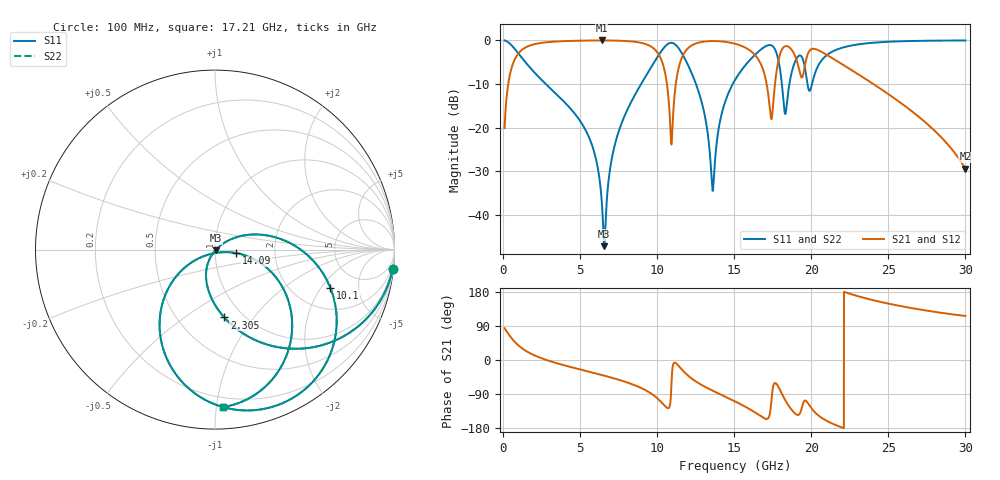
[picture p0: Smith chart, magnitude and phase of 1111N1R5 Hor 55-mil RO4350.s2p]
# GHz S MA R 50
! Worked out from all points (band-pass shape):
!   3201 points, 100 MHz to 30 GHz, reference 50 ohm
!   highest |S21| = -0.04 dB at 6.388 GHz (marker M1); lowest = -29.4 dB at 30 GHz (marker M2)
!   |S21| within 3 dB of the highest: 990.4 MHz to 10.07 GHz (9.075 GHz wide, 164 % of centre); 11.73 GHz to 16.26 GHz (4.523 GHz wide, 32.3 % of centre)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
!   lowest |S11| = -47.1 dB at 6.566 GHz (marker M3), VSWR 1.01, Z = 50.3 - j0.308 ohm
!   |S11| at or under -10 dB: 2.772 GHz to 8.957 GHz (6.185 GHz wide, 105 % of centre); 12.52 GHz to 14.91 GHz (2.388 GHz wide, 17.4 % of centre); 18.09 GHz to 18.58 GHz (487.3 MHz wide, 2.66 % of centre)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
!   |S22| runs from -47.1 to 0.0 dB; largest |S21 - S12| = 0
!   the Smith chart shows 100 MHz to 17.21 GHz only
!   S11 on the Smith chart (normalised r, x): 100 MHz: 1, -18; 2.305 GHz: 0.82, -0.73; 10.1 GHz: 3.13, -2.46; 14.09 GHz: 1.27, -0.05; 17.21 GHz: 0.14, -1.05
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0.1  0.9951 -6.3  0.09907 83.7  0.09907 83.7  0.9951 -6.3
0.7447187  0.8017 -41.5  0.5969 48.5  0.5969 48.5  0.8017 -41.5
2.305125  0.3818 -82.2  0.9223 7.6  0.9223 7.6  0.3818 -82.2
5.089563  0.1131 -114.3  0.9899 -25.9  0.9899 -25.9  0.1131 -114.3
6.388344  0.01562 -113.7  0.9949 -39.4  0.9949 -39.4  0.01562 -113.7
6.565875  0.00443 -43.7  0.9948 -41.3  0.9948 -41.3  0.00443 -43.7
7.472219  0.08737 34.4  0.9894 -51.7  0.9894 -51.7  0.08737 34.4
10.06978  0.6651 -17.1  0.7024 -103.3  0.7024 -103.3  0.6651 -17.1
10.09781  0.6769 -18.3  0.6897 -104.4  0.6897 -104.4  0.6769 -18.3
10.92941  0.9345 -66.9  0.06459 -61.4  0.06459 -61.4  0.9345 -66.9
11.84509  0.5926 -120.3  0.754 -35.3  0.754 -35.3  0.5926 -120.3
13.58303  0.01963 -94.7  0.9795 -80.7  0.9795 -80.7  0.01963 -94.7
14.08759  0.121 -9.3  0.9727 -90.5  0.9727 -90.5  0.121 -9.3
15.05  0.3512 -22.8  0.9129 -109.2  0.9129 -109.2  0.3512 -22.8
17.20841  0.8779 -87.0  0.2395 -153.4  0.2395 -153.4  0.8779 -87.0
17.79706  0.6631 -129.4  0.5047 -66.2  0.5047 -66.2  0.6631 -129.4
18.31097  0.1435 -99.4  0.8554 -106.1  0.8554 -106.1  0.1435 -99.4
19.16125  0.6573 -82.7  0.5048 -145.0  0.5048 -145.0  0.6573 -82.7
20.03956  0.3125 -71.3  0.7953 -128.9  0.7953 -128.9  0.3125 -71.3
21.95503  0.8167 -90.1  0.5388 -177.6  0.5388 -177.6  0.8167 -90.1
25.01978  0.9618 -122.8  0.2412 148.6  0.2412 148.6  0.9618 -122.8
30  0.9946 -156.5  0.03398 116.4  0.03398 116.4  0.9946 -156.5
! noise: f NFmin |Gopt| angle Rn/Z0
0.1  0.002042  0.9233  2.945  0.005891
3.417  0.01224  0.5624  24.44  0.004822
6.743  0.02418  0.5688  42.24  0.00891
10.06  0.1025  0.8289  60.69  0.09423
13.39  0.06752  0.6855  80.12  0.02501
16.7  0.2093  0.8635  96.24  0.1477
20.03  0.2623  0.8689  113.4  0.1314
23.35  0.1711  0.7951  125.2  0.03833
26.67  0.3142  0.885  140.6  0.06956
30  1.153  0.9683  157.2  0.3275
